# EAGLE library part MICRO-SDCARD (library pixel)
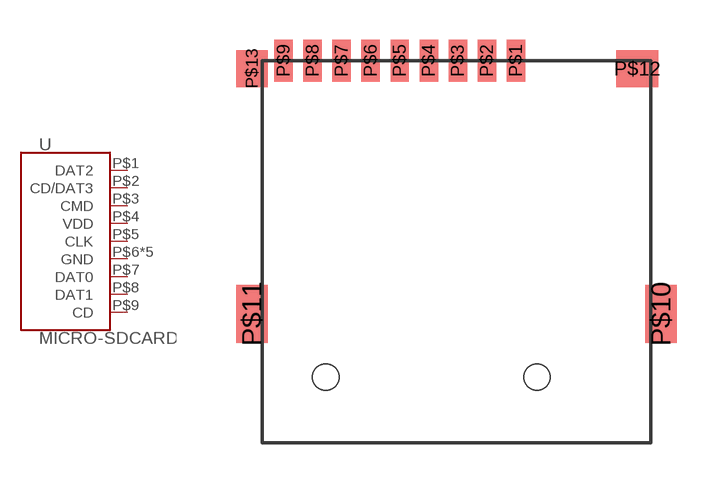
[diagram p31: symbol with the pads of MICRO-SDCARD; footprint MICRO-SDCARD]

Designator prefix -

## MICRO-SDCARD  [MICRO-SDCARD]
P$1  DAT2
P$2  CD/DAT3
P$3  CMD
P$4  VDD  pwr
P$5  CLK
P$6  GND  pwr
P$7  DAT0
P$8  DAT1
P$9  CD
P$10  GND  pwr
P$11  GND  pwr
P$12  GND  pwr
P$13  GND  pwr

## Footprint MICRO-SDCARD (pad centres in mm)
smd 0.7 x 1.6: P$1 2.25,0; P$2 1.15,0; P$3 0.05,0; P$4 -1.05,0; P$5 -2.15,0; P$6 -3.25,0; P$7 -4.35,0; P$8 -5.45,0; P$9 -6.55,0
smd 1.2 x 2.2: P$10 7.75,-9.6; P$11 -7.75,-9.6
smd 1.6 x 1.4: P$12 6.85,-0.3
smd 1.2 x 1.4: P$13 -7.75,-0.3
hole 1 at -4.95,-12
hole 1 at 3.05,-12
